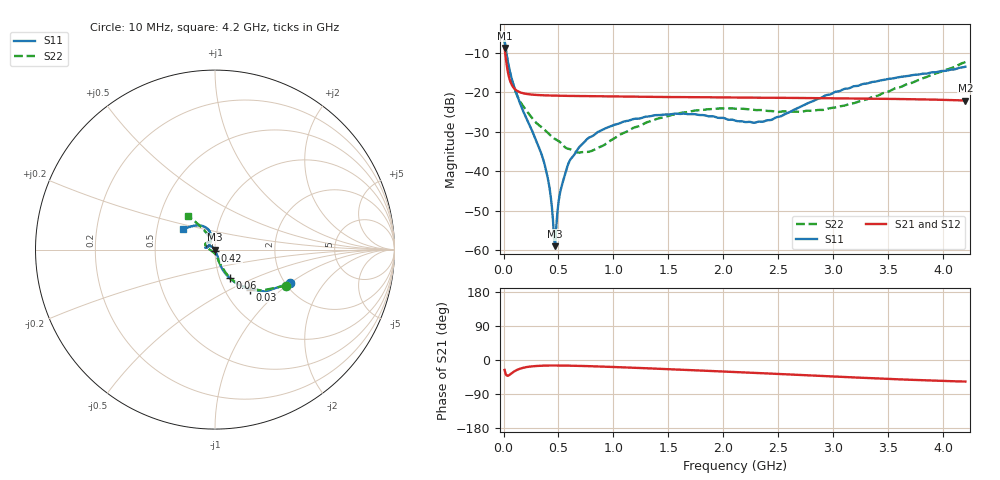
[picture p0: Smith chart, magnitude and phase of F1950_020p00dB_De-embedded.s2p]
! Integrated Device Technology
! Corporate Headquarters
! 6024 Silver Creek Valley Road
! San Jose, CA 95138  USA
! Phone:  1-408-284-8200
! Toll Free:  1-800-223-1366
! Webpage:  http://www.idt.com/
! Timing and RF Division
! 515 Groton Road, Suite 102
! Westford, MA 01886-6024
! Device:  F1950
! Description: 7-bit 0.25 dB Digital Step Attenuator
! Frequency:  150.0 -  4000.00 MHz
! Package:  4x4 mm Thin QFN Plastic Package: 24 pin
! Ports:  2 RF, 12 DC
!  Pin  1  = D0
!  Pin  2  = VDD
!  Pin  3  = Vmode
!  Pin  4  = GND
!  Pin  5  = RF1  =  Port 1
!  Pin  6  = GND
!  Pin  7  = GND
!  Pin  8  = GND
!  Pin  9  = GND
!  Pin 10  = GND
!  Pin 11  = GND
!  Pin 12  = GND
!  Pin 13  = GND
!  Pin 14  = RF2  =  Port 2
!  Pin 15  = GND
!  Pin 16  = LE
!  Pin 17  = CLK
!  Pin 18  = DATE
!  Pin 19  = D6
!  Pin 20  = D5
!  Pin 21  = D4
!  Pin 22  = D3
!  Pin 23  = D2
!  Pin 24  = D1
! State:  80
! Atten State:  20.00 dB
! Voltage:  +5.00 Volts
! Current:  Not Measured mA
! Data:  The device was measured on a the F195X evaluation board which has
!  individual transmission lines to the RF pins.  Data was collected
!  using a calibrated network analyzer.  The evaluation board was
!  de-embedded using a TRL calibration technique.
!  The reference plane is the edge of the package pin.
! Misc:  Board 2019
!  Action Tracker AT0250
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# GHz S dB R 50
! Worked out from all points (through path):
!   420 points, 10 MHz to 4.2 GHz, reference 50 ohm
!   highest |S21| = -8.72 dB at 10 MHz (marker M1); lowest = -22.0 dB at 4.2 GHz (marker M2)
!   group delay of S21, straight-line fit = 29.1 ps
!   lowest |S11| = -59.0 dB at 470 MHz (marker M3), VSWR 1.00, Z = 49.9 - j0.0164 ohm
!   |S11| at or under -10 dB: 26.96 MHz to end of sweep
!   |S22| runs from -35.2 to -7.1 dB; largest |S21 - S12| = 0.00015
!   S11 on the Smith chart (normalised r, x): 10 MHz: 2.10, -1.00; 30 MHz: 1.31, -0.64; 60 MHz: 1.12, -0.37; 420 MHz: 1.00, -0.01; 4.2 GHz: 0.68, +0.17
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0.01  -6.82 -24.3  -8.72 -26.2  -8.72 -26.2  -7.06 -26.9
0.03  -10.55 -48.8  -13.22 -41.2  -13.22 -41.2  -11.02 -49.8
0.06  -14.94 -62.6  -17.06 -38.2  -17.06 -38.2  -15.13 -62.3
0.11  -19.60 -70.3  -19.32 -28.0  -19.32 -28.0  -19.87 -67.9
0.17  -24.16 -71.0  -20.14 -21.2  -20.14 -21.2  -23.13 -72.1
0.35  -36.02 -67.6  -20.70 -15.0  -20.70 -15.0  -28.88 -78.5
0.42  -44.42 -73.9  -20.77 -14.6  -20.77 -14.6  -30.69 -80.8
0.45  -52.41 -88.8  -20.79 -14.5  -20.79 -14.5  -31.45 -84.6
0.47  -58.96 -171.6  -20.81 -14.5  -20.81 -14.5  -31.81 -87.5
0.48  -54.01 155.6  -20.81 -14.5  -20.81 -14.5  -31.97 -88.6
0.52  -44.69 138.9  -20.83 -14.5  -20.83 -14.6  -32.72 -91.2
0.57  -39.68 134.0  -20.86 -14.7  -20.86 -14.7  -34.08 -99.0
0.61  -36.90 136.0  -20.88 -14.9  -20.88 -15.0  -34.42 -106.9
0.71  -33.25 137.7  -20.91 -15.7  -20.91 -15.7  -35.13 -125.7
0.99  -28.40 147.8  -21.01 -18.3  -21.01 -18.4  -31.92 -172.1
1.41  -25.73 163.9  -21.13 -23.1  -21.12 -23.1  -26.57 165.3
1.73  -25.48 169.5  -21.19 -27.0  -21.19 -27.0  -24.63 156.6
2.11  -27.15 159.5  -21.28 -31.9  -21.28 -32.0  -24.13 147.1
2.43  -26.99 127.6  -21.34 -35.9  -21.34 -35.9  -24.69 137.2
2.81  -22.25 105.9  -21.42 -41.0  -21.42 -41.0  -24.67 122.1
3.51  -16.53 118.0  -21.62 -50.0  -21.61 -50.0  -19.67 117.2
4.2  -13.47 146.3  -22.04 -56.9  -22.03 -57.0  -12.29 128.7
